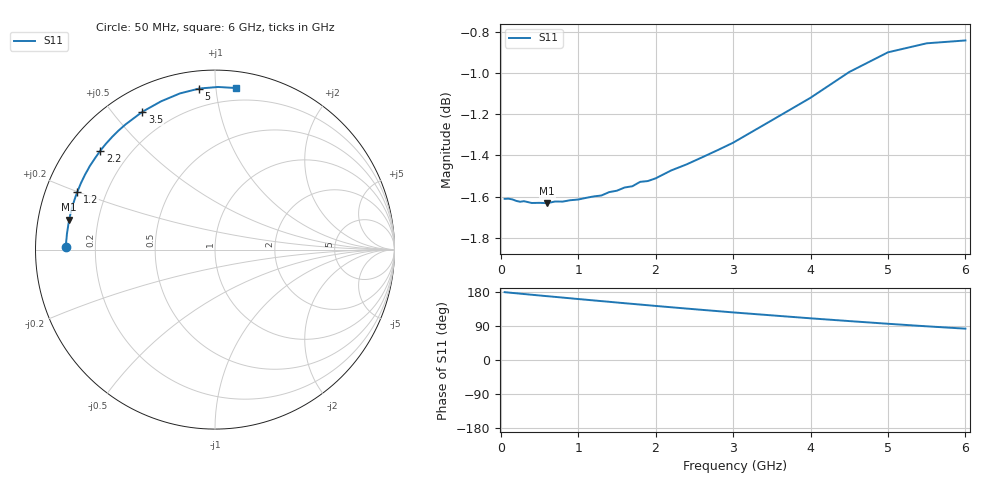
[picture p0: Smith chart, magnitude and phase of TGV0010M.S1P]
! SIEMENS Discrete & RF Semiconductors
! BAT64
! Si Schottky Diode in SOT23
! IF = 10 mA
! S-Parameters:  February  1997
# GHz  S  MA  R  50
!  f  S11
! GHz  MAG  ANG
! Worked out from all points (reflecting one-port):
!   34 points, 50 MHz to 6 GHz, reference 50 ohm
!   lowest |S11| = -1.6 dB at 600 MHz (marker M1), VSWR 10.67, Z = 4.73 + j5.03 ohm
!   phase of S11 starts at 179 deg and turns -96 deg over the sweep
!   S11 on the Smith chart (normalised r, x): 50 MHz: 0.09, +0.01; 1.2 GHz: 0.10, +0.20; 2.2 GHz: 0.10, +0.37; 3.5 GHz: 0.10, +0.60; 5 GHz: 0.09, +0.90; 6 GHz: 0.11, +1.13
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0.05  0.8307 179.0
0.15  0.8304 177.0
0.2  0.8297 176.1
0.3  0.8296 174.1
0.5  0.8288 170.3
0.6  0.8287 168.4
0.7  0.8294 166.6
0.8  0.8294 164.7
0.9  0.83 162.8
1  0.8304 160.9
1.1  0.8311 159.1
1.2  0.8318 157.2
1.4  0.8338 153.6
1.5  0.8345 151.7
1.6  0.836 149.9
1.8  0.8386 146.3
2  0.8403 142.7
2.2  0.844 139.2
2.4  0.8469 135.7
2.6  0.8502 132.3
2.8  0.8536 129.0
3  0.8572 125.6
3.5  0.868 117.8
4  0.879 110.0
4.5  0.8918 102.7
5  0.9017 95.6
5.5  0.9062 88.9
6  0.9077 82.7
